PROGRAM MAIN
VAR
	count1: FB_Count; 
	count2: FB_CountEX; 
	icount: I_Count;
	i,k :INT;
	Startcount:BOOL;
	check: BOOL;
	max_i: INT;
	max_k: INT;
	change: BOOL:=TRUE;
END_VAR

IF change THEN
	icount:=count1;
ELSE
	icount:=count2;
	check:=count2.M_Check(bCheckValue:=Startcount );
END_IF
				
icount.M_Count( bEnable:=Startcount ,
	            i_Wert=>i,
				k_Wert=>k );

icount.P_Max_i:=1000;
max_i:=icount.P_Max_i;

icount.P_Max_k:=2000;
max_k:=icount.P_Max_k;

END_PROGRAM
